| TEXAS INSTRUMENTS INCORPORATED
| Standard Linear and Logic Group
| IBIS Model of SN74LVC161284
| 19-BIT BUS INTERFACE
| This file contains package information for the following:
|  TSSOP 48-pin (DGG) package as [Component] LVC161284_DGG
|  SSOP 48-pin (DL) package as [Component] LVC161284_DL
| This device can be powered at the following Vccs:
|  3.3 volt Vcc
| This file provides unique models under the [Model Selector] for each mode.
| For operation at a specific mode, select the appropriate model after each
| [Model Selector] keyword.
[IBIS Ver]   3.2
[Comment char]  |_char
[File Name]   sn74lvc161284.ibs
[File Rev]   1.1 | a_die
[Date]   October 17, 2002
[Source]   Data created from TI-SPICE simulations at TI-SLL.
[Notes]   The following is an IBIS list for the LVC161284.
   Please contact sllibis@ti.com with questions and
   comments concerning SLL IBIS models.
   End point warning due to DC and AC data Mismatch
   The warning typ/min/max values never become zero- due to
   presence of pullup-resistor.
   Non-monotonic data due to PMOS transistor connected to
   VCC CABLE.
   VCC CABLE was equal to VCC during measurement.
   Measurement method of C_comp in IBIS and Ci/Cio in datasheet
   is not same
   Power Clamp data deleted from control input model as there
   is no power-clamp diode.
[Disclaimer] Property of Texas Instruments Incorporated.  Unauthorized
   reproduction and/or distribution is strictly prohibited.
   This product is protected under copyright law.
   Created  2002, (C) Copyright  2002, Texas Instruments
   Incorporated, All Rights Reserved
   UNLESS THERE IS A SIGNED, WRITTEN AGREEMENT TO THE
   CONTRARY, TEXAS INSTRUMENTS (TI) IS PROVIDING THE IBIS
   MODELS  AND WITHOUT ANY WARRANTY, EXPRESSED OR
   IMPLIED.  TI assumes no liability for:
   1) the accuracy of the IBIS models provided to your
   company;
   2) the proper functioning of these IBIS Models in your
   design or for any resulting applications; or
   3) infringement of patents, copyrights or intellectual
   property rights resulting from your use of these IBIS
   models.
   TI provides IBIS Models as a service to our customers.
   You and your company shall not distribute, sell or give
   these models to anyone else without prior written
   permission from TI.
   TI reserves the right to make changes to our products or
   to discontinue any semiconductor product or service
   without notice, and advises our customers to obtain the
   latest version of relevant information to verify, before
   placing orders, that the information being relied on is
   current.
   Please be aware that your receipt and use of the IBIS
   information provided shall serve as acceptance of these
   terms and conditions.  If you do not accept these terms,
   you should return or destroy the IBIS models and any
   other accompanying information immediately.
| Component LVC161284_DGG 48-pin TSSOP
[Component]   LVC161284_DGG
[Manufacturer]   Texas Instruments, Inc.
[Package]
|   typ   min   max
R_pkg   4.400e-02   3.800e-02   5.100e-02
L_pkg   3.019e-09   2.486e-09   4.099e-09
C_pkg   5.070e-13   3.340e-13   8.090e-13
[Pin]   signal_name   model_name   R_pin   L_pin   C_pin
1   HD   LVC161284_HD   4.100e-02   4.017e-09   7.590e-13
2   A9   LVC161284_AIN   4.200e-02   3.737e-09   7.920e-13
3   A10   LVC161284_AIN   4.200e-02   3.480e-09   6.610e-13
4   A11   LVC161284_AIN   3.800e-02   3.131e-09   5.750e-13
5   A12   LVC161284_AIN   4.700e-02   3.122e-09   5.660e-13
6   A13   LVC161284_AIN   4.300e-02   2.948e-09   5.040e-13
7   VCC   POWER   4.500e-02   2.845e-09   3.970e-13
8   A1   LVC161284_AIO   4.900e-02   2.835e-09   3.940e-13
9   A2   LVC161284_AIO   4.800e-02   2.715e-09   3.780e-13
10   GND   GND   5.000e-02   2.664e-09   3.630e-13
11   A3   LVC161284_AIO   5.000e-02   2.585e-09   3.480e-13
12   A4   LVC161284_AIO   4.900e-02   2.550e-09   3.370e-13
13   A5   LVC161284_AIO   4.900e-02   2.541e-09   3.360e-13
14   A6   LVC161284_AIO   5.000e-02   2.574e-09   3.480e-13
15   GND   GND   4.900e-02   2.618e-09   3.590e-13
16   A7   LVC161284_AIO   4.600e-02   2.671e-09   3.750e-13
17   A8   LVC161284_AIO   4.500e-02   2.754e-09   3.890e-13
18   VCC   POWER   4.400e-02   2.823e-09   4.500e-13
19   PERI_IN   LVC161284_PIN   4.200e-02   2.968e-09   5.030e-13
20   A14   LVC161284_AOUT   5.100e-02   3.108e-09   5.350e-13
21   A15   LVC161284_AOUT   4.200e-02   3.175e-09   5.870e-13
22   A16   LVC161284_AOUT   4.100e-02   3.449e-09   6.780e-13
23   A17   LVC161284_AOUT   4.400e-02   3.766e-09   8.040e-13
24   HOST_OUT   LVC161284_HOUT   4.300e-02   4.065e-09   7.610e-13
25   HOST_IN   LVC161284_HIN   4.100e-02   3.994e-09   7.570e-13
26   C17   LVC161284_CIN   3.900e-02   3.649e-09   7.890e-13
27   C16   LVC161284_CIN   3.800e-02   3.362e-09   6.600e-13
28   C15   LVC161284_CIN   3.800e-02   3.082e-09   5.740e-13
29   C14   LVC161284_CIN   4.400e-02   2.990e-09   5.220e-13
30   PERI_OUT   LVC161284_POUT   4.100e-02   2.917e-09   4.950e-13
31   VCC_CABLE  POWER   4.300e-02   2.820e-09   4.480e-13
32   B8   LVC161284_BIO   4.300e-02   2.699e-09   3.850e-13
33   B7   LVC161284_BIO   4.500e-02   2.628e-09   3.720e-13
34   GND   GND   4.600e-02   2.556e-09   3.560e-13
35   B6   LVC161284_BIO   4.600e-02   2.495e-09   3.440e-13
36   B5   LVC161284_BIO   4.700e-02   2.487e-09   3.340e-13
37   B4   LVC161284_BIO   4.700e-02   2.490e-09   3.350e-13
38   B3   LVC161284_BIO   4.600e-02   2.486e-09   3.430e-13
39   GND   GND   4.500e-02   2.566e-09   3.560e-13
40   B2   LVC161284_BIO   4.400e-02   2.639e-09   3.740e-13
41   B1   LVC161284_BIO   4.300e-02   2.701e-09   3.860e-13
42   VCC_CABLE  POWER   4.300e-02   2.817e-09   4.500e-13
43   Y13   LVC161284_YOUT   4.100e-02   2.935e-09   5.010e-13
44   Y12   LVC161284_YOUT   4.700e-02   3.035e-09   5.290e-13
45   Y11   LVC161284_YOUT   4.300e-02   3.171e-09   5.890e-13
46   Y10   LVC161284_YOUT   4.000e-02   3.415e-09   6.820e-13
47   Y9   LVC161284_YOUT   4.300e-02   3.741e-09   8.090e-13
48   DIR   LVC161284_DIR   4.400e-02   4.099e-09   7.640e-13
| Component LVC161284_DL 48-pin SSOP
[Component]   LVC161284_DL
[Manufacturer]   Texas Instruments, Inc.
[Package]
|   typ   min   max
R_pkg   4.800e-02   3.800e-02   5.300e-02
L_pkg   6.046e-09   5.084e-09   7.968e-09
C_pkg   8.130e-13   5.690e-13   1.157e-12
[Pin]   signal_name   model_name   R_pin   L_pin   C_pin
1   HD   LVC161284_HD   4.600e-02   7.968e-09   1.017e-12
2   A9   LVC161284_AIN   4.400e-02   7.299e-09   1.157e-12
3   A10   LVC161284_AIN   4.300e-02   6.765e-09   1.058e-12
4   A11   LVC161284_AIN   4.100e-02   6.269e-09   9.330e-13
5   A12   LVC161284_AIN   3.800e-02   5.856e-09   8.290e-13
6   A13   LVC161284_AIN   4.600e-02   5.802e-09   7.900e-13
7   VCC   POWER   5.000e-02   5.656e-09   7.380e-13
8   A1   LVC161284_AIO   5.300e-02   5.500e-09   6.430e-13
9   A2   LVC161284_AIO   5.200e-02   5.304e-09   6.060e-13
10   GND   GND   5.300e-02   5.189e-09   5.830e-13
11   A3   LVC161284_AIO   5.100e-02   5.084e-09   5.690e-13
12   A4   LVC161284_AIO   5.300e-02   5.862e-09   8.330e-13
13   A5   LVC161284_AIO   5.300e-02   5.862e-09   8.330e-13
14   A6   LVC161284_AIO   5.100e-02   5.084e-09   5.690e-13
15   GND   GND   5.300e-02   5.189e-09   5.830e-13
16   A7   LVC161284_AIO   5.200e-02   5.304e-09   6.060e-13
17   A8   LVC161284_AIO   5.300e-02   5.500e-09   6.430e-13
18   VCC   POWER   5.000e-02   5.656e-09   7.380e-13
19   PERI_IN   LVC161284_PIN   4.600e-02   5.802e-09   7.900e-13
20   A14   LVC161284_AOUT   3.800e-02   5.856e-09   8.290e-13
21   A15   LVC161284_AOUT   4.100e-02   6.269e-09   9.330e-13
22   A16   LVC161284_AOUT   4.300e-02   6.765e-09   1.058e-12
23   A17   LVC161284_AOUT   4.400e-02   7.299e-09   1.157e-12
24   HOST_OUT   LVC161284_HOUT   4.600e-02   7.968e-09   1.017e-12
25   HOST_IN   LVC161284_HIN   4.600e-02   7.968e-09   1.017e-12
26   C17   LVC161284_CIN   4.400e-02   7.299e-09   1.157e-12
27   C16   LVC161284_CIN   4.300e-02   6.765e-09   1.058e-12
28   C15   LVC161284_CIN   4.100e-02   6.269e-09   9.330e-13
29   C14   LVC161284_CIN   3.800e-02   5.856e-09   8.290e-13
30   PERI_OUT   LVC161284_POUT   4.600e-02   5.802e-09   7.900e-13
31   VCC_CABLE  POWER   5.000e-02   5.656e-09   7.380e-13
32   B8   LVC161284_BIO   5.300e-02   5.500e-09   6.430e-13
33   B7   LVC161284_BIO   5.200e-02   5.304e-09   6.060e-13
34   GND   GND   5.300e-02   5.189e-09   5.830e-13
35   B6   LVC161284_BIO   5.100e-02   5.084e-09   5.690e-13
36   B5   LVC161284_BIO   5.300e-02   5.862e-09   8.330e-13
37   B4   LVC161284_BIO   5.300e-02   5.862e-09   8.330e-13
38   B3   LVC161284_BIO   5.100e-02   5.084e-09   5.690e-13
39   GND   GND   5.300e-02   5.189e-09   5.830e-13
40   B2   LVC161284_BIO   5.200e-02   5.304e-09   6.060e-13
41   B1   LVC161284_BIO   5.300e-02   5.500e-09   6.430e-13
42   VCC_CABLE  POWER   5.000e-02   5.656e-09   7.380e-13
43   Y13   LVC161284_YOUT   4.600e-02   5.802e-09   7.900e-13
44   Y12   LVC161284_YOUT   3.800e-02   5.856e-09   8.290e-13
45   Y11   LVC161284_YOUT   4.100e-02   6.269e-09   9.330e-13
46   Y10   LVC161284_YOUT   4.300e-02   6.765e-09   1.058e-12
47   Y9   LVC161284_YOUT   4.400e-02   7.299e-09   1.157e-12
48   DIR   LVC161284_DIR   4.600e-02   7.967e-09   1.017e-12
| Model LVC161284_BIO
[Model Selector]   LVC161284_BIO
LVC161284_BIO_OD   Open-Drain Mode
LVC161284_BIO_TP   Totem-Pole Mode
| Model LVC161284_YOUT_OD
[Model Selector]   LVC161284_YOUT
LVC161284_YOUT_OD   Open-Drain Mode
LVC161284_YOUT_TP   Totem-Pole Mode
| Model LVC161284_POUT
[Model Selector]   LVC161284_POUT
LVC161284_POUT_OD   Open-Drain Mode
LVC161284_POUT_TP   Totem-Pole Mode
| Models and submodels in the file (15): LVC161284_DIR (Input), LVC161284_PIN (Input), LVC161284_AIN (Input), LVC161284_HD (Input), LVC161284_HIN (Input), LVC161284_CIN (Input), LVC161284_AIO (I/O), LVC161284_BIO_OD (I/O_open_drain), LVC161284_AOUT (Output), LVC161284_HOUT (Output), LVC161284_YOUT_OD (Open_drain), LVC161284_POUT_OD (Open_drain), LVC161284_POUT_TP (Output), LVC161284_YOUT_TP (3-state), LVC161284_BIO_TP (I/O)
